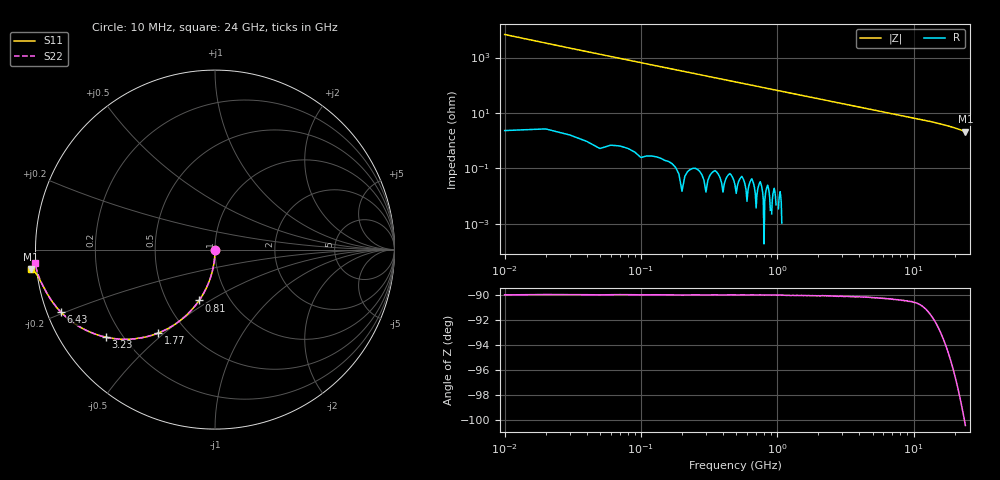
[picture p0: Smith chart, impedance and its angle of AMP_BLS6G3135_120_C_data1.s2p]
! Created Mon May 10 11:39:28 2010
# ghz S ma R 50
! 2 Port Network Data from SP1.SP block
! freq  magS11  angS11  magS21  angS21  magS12  angS12  magS22  angS22
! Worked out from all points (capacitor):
!   2400 points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, 10 MHz to 24 GHz, reference 50 ohm
!   read as one part in shunt: C = 2.45 pF near 130 MHz
!   lowest |Z| = 2.11 ohm at 24 GHz (marker M1)
!   S11 on the Smith chart (normalised r, x): 10 MHz: 1.00, -0.01; 810 MHz: 0.72, -0.45; 1.77 GHz: 0.35, -0.48; 3.23 GHz: 0.14, -0.35; 6.43 GHz: 0.04, -0.19; 24 GHz: -0.02, -0.05
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0.01  0.003601 -89.9  1 -0.2  1 -0.2  0.0037 -89.9
0.07  0.02655 -91.5  0.9996 -1.5  0.9996 -1.5  0.02697 -91.5
0.15  0.05692 -93.3  0.9983 -3.3  0.9983 -3.3  0.05758 -93.3
0.19  0.07271 -94.2  0.9973 -4.2  0.9973 -4.2  0.07278 -94.2
0.25  0.09498 -95.5  0.9954 -5.5  0.9954 -5.5  0.0956 -95.5
0.35  0.1326 -97.7  0.991 -7.7  0.991 -7.7  0.1333 -97.7
0.48  0.1811 -100.5  0.9833 -10.5  0.9833 -10.5  0.1813 -100.5
0.63  0.2349 -103.6  0.9718 -13.6  0.9718 -13.6  0.2352 -103.6
0.81  0.297 -107.3  0.9547 -17.3  0.9547 -17.3  0.297 -107.3
1.01  0.3615 -111.2  0.9322 -21.3  0.9322 -21.3  0.3615 -111.2
1.23  0.4274 -115.3  0.9041 -25.3  0.9041 -25.3  0.4269 -115.3
1.77  0.5623 -124.2  0.827 -34.3  0.827 -34.3  0.5618 -124.2
2.41  0.6791 -132.8  0.7343 -42.9  0.7343 -42.9  0.6787 -132.8
3.23  0.778 -141.2  0.6285 -51.3  0.6285 -51.3  0.7779 -141.1
4.01  0.8381 -147.1  0.5459 -57.2  0.5459 -57.2  0.8379 -147.0
5.08  0.8897 -152.9  0.458 -63.1  0.458 -63.1  0.8892 -152.8
6.43  0.9266 -158.0  0.3779 -68.2  0.3779 -68.2  0.9262 -157.9
8.01  0.9506 -162.1  0.3125 -72.4  0.3125 -72.4  0.9503 -161.9
12.01  0.9787 -168.0  0.215 -78.9  0.215 -78.9  0.9782 -167.8
16.01  0.9969 -171.3  0.1568 -84.5  0.1568 -84.5  0.9928 -171.3
20.01  1.014 -173.1  0.1165 -89.8  0.1165 -89.8  1.001 -173.8
24  1.032 -173.9  0.08597 -95.2  0.08597 -95.2  1.005 -175.7
